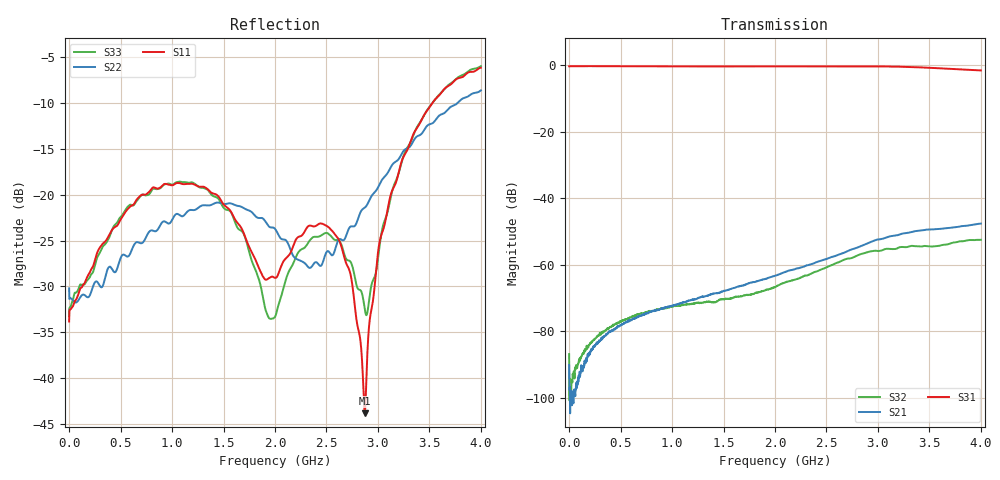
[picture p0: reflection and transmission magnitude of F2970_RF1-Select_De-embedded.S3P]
! Integrated Device Technology
! Corporate Headquarters
! 6024 Silver Creek Valley Road
! San Jose, CA 95138  USA
! Phone:  1-408-284-8200
! Toll Free:  1-800-223-1366
! Webpage:  http://www.idt.com/
! Timing and RF Division
! 515 Groton Road, Suite 102
! Westford, MA 01886-6024
! Device:  F2970
! Description: 75 Ohm SP2T RF Switch
! Frequency:  5.0 -  3000.00 MHz
! Package:  4x4 mm LQFN Plastic Package: 20 pin
! Ports:  3 RF, 2 DC
!  Pin  1  = GND
!  Pin  2  = GND
!  Pin  3  = RF1  = Port 1
!  Pin  4  = GND
!  Pin  5  = GND
!  Pin  6  = GND
!  Pin  7  = GND
!  Pin  8  = RFC  = Port 3
!  Pin  9  = GND
!  Pin 10  = GND
!  Pin 11  = GND
!  Pin 12  = GND
!  Pin 13  = RF2  = Port 2
!  Pin 14  = GND
!  Pin 15  = GND
!  Pin 16  = C2
!  Pin 17  = C1
!  Pin 18  = GND
!  Pin 19  = GND
!  Pin 20  = VCC
! State:  RF1 Selected
! Voltage:  Vcc = +3.0 Volts
!  C1 = 0.0 V,  C2 = 0.0 V
! Data:  The device was measured on a the F2970 evaluation board which has
!  individual transmission lines to the RF pins.  Data was collected
!  using a calibrated network analyzer.  The evaluation board was
!  de-embedded using a PORT EXTENSTION technique.
!  The reference plane is the edge of the package pin.
! Misc:
!  Action Tracker AT0363
! Date Measured:  2014-11-08
! Date:  2016-11-29  MJV
! Note:
!  Integrated Device Technology supplies this data as a sample of measured
!  data at the package pin for this product.  Your particular data for this
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# Hz S dB R 75
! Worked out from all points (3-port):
!   1601 points, 300 kHz to 4 GHz, reference 75 ohm
!   strongest paths, dB at 300 kHz, 1 GHz, 2 GHz, 3 GHz, 4 GHz:
!     S31: -0.3, -0.3, -0.3, -0.3, -1.5
!     S21: -90.0, -72.3, -63.3, -52.3, -47.6
!     S32: -86.8, -72.5, -66.6, -55.8, -52.4
!   lowest |S11| = -43.8 dB at 2.873 GHz (marker M1), VSWR 1.01, Z = 75.6 - j0.75 ohm
!   |S11| at or under -10 dB: start of sweep to 3.531 GHz
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300000  -33.83 28.1  -95.35 -179.1  -0.27 0.7
        -90.02 63.4  -30.22 167.7  -95.42 97.9
        -0.26 0.6  -86.81 7.5  -33.21 5.4
1.077719e9  -18.76 -91.6  -71.48 120.6  -0.30 -13.5
            -71.57 121.4  -22.27 -91.1  -72.14 105.8
            -0.31 -13.5  -72.23 105.9  -18.59 -94.2
1.570182e9  -21.82 -85.4  -67.26 140.5  -0.30 -19.3
            -67.21 140.1  -20.96 -74.6  -70.12 131.7
            -0.30 -19.3  -70.15 131.8  -21.88 -94.3
2.00015e9  -29.07 -9.1  -63.23 154.7  -0.29 -24.7
           -63.28 154.9  -23.73 -68.4  -66.65 159.5
           -0.29 -24.6  -66.64 159.3  -33.33 -4.6
2.590106e9  -24.43 39.5  -57.24 167.1  -0.29 -32.1
            -57.25 167.1  -25.72 -139.0  -59.51 174.4
            -0.29 -32.0  -59.50 174.4  -24.96 31.7
2.740094e9  -29.04 34.6  -55.38 168.0  -0.28 -34.1
            -55.37 168.0  -23.46 -148.5  -57.95 171.7
            -0.29 -34.1  -57.97 171.6  -27.45 15.8
2.872585e9  -43.83 -50.4  -53.88 167.5  -0.28 -36.1
            -53.86 167.7  -21.41 -158.5  -56.42 168.9
            -0.29 -36.0  -56.42 168.8  -32.52 -26.4
3.010074e9  -25.55 -125.9  -52.31 162.5  -0.29 -38.3
            -52.32 162.6  -19.01 -165.1  -55.83 163.2
            -0.30 -38.3  -55.81 162.9  -26.11 -106.7
3.235057e9  -16.22 -136.7  -50.61 157.3  -0.40 -42.2
            -50.60 157.4  -15.47 -165.1  -54.60 158.7
            -0.41 -42.1  -54.60 158.8  -16.26 -127.8
4e9  -6.17 -140.1  -47.55 147.0  -1.50 -50.7
     -47.55 147.1  -8.65 -139.1  -52.44 157.7
     -1.51 -50.5  -52.44 157.9  -6.01 -135.9
